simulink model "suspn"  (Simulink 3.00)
settings: Solver=ode45  SolverMode=SingleTasking  StartTime=0.0  StopTime=10  MaxStep=0.01  RelTol=1e-3  AbsTol=1e-6
PreLoadFcn:
  | suspdat
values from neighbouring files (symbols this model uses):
  cf = 2500    [suspdat.m]
  cr = 2000    [suspdat.m]
  Iyy = 2100    [suspdat.m]
  kf = 28000    [suspdat.m]
  kr = 21000    [suspdat.m]
  Lf = 0.9    [suspdat.m]
  Lr = 1.2    [suspdat.m]
  Mb = 1200    [suspdat.m]

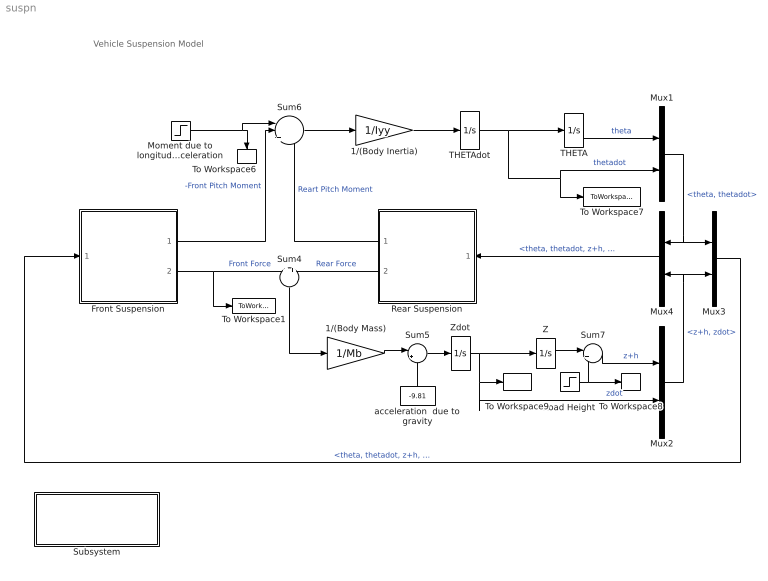
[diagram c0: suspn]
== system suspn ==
  note: Vehicle Suspension Model
  1/(Body Inertia) : Gain  Gain=1/Iyy  SaturateOnIntegerOverflow=on
  1/(Body Mass) : Gain  Gain=1/Mb  SaturateOnIntegerOverflow=on
  Front Suspension : Subsystem  mask(half-car suspension){K=kf, C=cf, L=-Lf}
      mask prompts: K "Stiffness = spring rate:"; C "Damping rate:"; L "Moment arm:"
      mask help: Half-Car Suspension The spring and damping rates for an individual wheel are entered below. Their combined effect as applied to two wheels at the specified distance from the center of mass is computed. The distance should be specified as positive if the subsystem is oriented such that increasing z corresponds to increasing theta, negative otherwise.
  Moment due to longitudinal vehicle acceleration : Step  Time=3  Before=0  After=100  SampleTime=0
  Mux1 : Mux  Inputs=2
  Mux2 : Mux  Inputs=2
  Mux3 : Mux  Inputs=2
  Mux4 : Mux  Orientation=left  Inputs=2
  Rear Suspension : Subsystem  Orientation=left  mask(half-car suspension){K=kr, C=cr, L=Lr}
      mask prompts: K "Stiffness = spring rate:"; C "Damping rate:"; L "Moment arm:"
      mask help: Half-Car Suspension The spring and damping rates for an individual wheel are entered below. Their combined effect as applied to two wheels at the specified distance from the center of mass is computed. The distance should be specified as positive if the subsystem is oriented such that increasing z corresponds to increasing theta, negative otherwise.
  Road Height : Step  Time=7  Before=0  After=0.01  SampleTime=0
  Subsystem : Subsystem
  Sum4 : Sum  Orientation=down  Inputs=++  SaturateOnIntegerOverflow=on
  Sum5 : Sum  Inputs=|++  SaturateOnIntegerOverflow=on
  Sum6 : Sum  Inputs=||+++  SaturateOnIntegerOverflow=on
  Sum7 : Sum  Inputs=|++  SaturateOnIntegerOverflow=on
  THETA : Integrator  ExternalReset=none  InitialConditionSource=internal  InitialCondition=-8.7e-20  LimitOutput=off  UpperSaturationLimit=inf  LowerSaturationLimit=-inf  ShowSaturationPort=off  ShowStatePort=off  AbsoluteTolerance=auto
  THETAdot : Integrator  ExternalReset=none  InitialConditionSource=internal  InitialCondition=8.04e-28  LimitOutput=off  UpperSaturationLimit=inf  LowerSaturationLimit=-inf  ShowSaturationPort=off  ShowStatePort=off  AbsoluteTolerance=auto
  To Workspace1 : ToWorkspace  VariableName=ForceF  SampleTime=0.01  SaveFormat=Matrix
  To Workspace6 : ToWorkspace  VariableName=Y  SampleTime=0.01  SaveFormat=Matrix
  To Workspace7 : ToWorkspace  VariableName=THETAdot  SampleTime=0.01  SaveFormat=Matrix
  To Workspace8 : ToWorkspace  VariableName=h  SampleTime=0.01  SaveFormat=Matrix
  To Workspace9 : ToWorkspace  VariableName=Zdot  SampleTime=0.01  SaveFormat=Matrix
  Z : Integrator  ExternalReset=none  InitialConditionSource=internal  InitialCondition=-0.12  LimitOutput=off  UpperSaturationLimit=inf  LowerSaturationLimit=-inf  ShowSaturationPort=off  ShowStatePort=off  AbsoluteTolerance=auto
  Zdot : Integrator  ExternalReset=none  InitialConditionSource=internal  InitialCondition=0  LimitOutput=off  UpperSaturationLimit=inf  LowerSaturationLimit=-inf  ShowSaturationPort=off  ShowStatePort=off  AbsoluteTolerance=auto
  acceleration  due to gravity : Constant  Orientation=up  Value=-9.81
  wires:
  Front Suspension/2(Vertical Force) -> Sum4/1, To Workspace1/1  "Front Force"
  Rear Suspension/2(Vertical Force) -> Sum4/2  "Rear Force"
  Sum4/1 -> 1/(Body Mass)/1
  Mux1/1 -> Mux3/1, Mux4/1  "<theta, thetadot>"
  Mux3/1 -> Front Suspension/1(THETA THETAdot Z Zdot)  "<theta, thetadot, z+h, zdot>"
  Mux4/1 -> Rear Suspension/1(THETA THETAdot Z Zdot)  "<theta, thetadot, z+h, zdot>"
  Sum5/1 -> Zdot/1
  acceleration  due to gravity/1 -> Sum5/2
  1/(Body Mass)/1 -> Sum5/1
  Z/1 -> Sum7/1
  Sum7/1 -> Mux2/1  "z+h"
  Zdot/1 -> Z/1, Mux2/2, To Workspace9/1  "zdot"
  Road Height/1 -> Sum7/2, To Workspace8/1
  Mux2/1 -> Mux3/2, Mux4/2  "<z+h, zdot>"
  Moment due to longitudinal vehicle acceleration/1 -> To Workspace6/1, Sum6/1
  Sum6/1 -> 1/(Body Inertia)/1
  Rear Suspension/1(pitch Torque) -> Sum6/3  "Reart Pitch Moment"
  Front Suspension/1(pitch Torque) -> Sum6/2  "-Front Pitch Moment"
  1/(Body Inertia)/1 -> THETAdot/1
  THETA/1 -> Mux1/1  "theta"
  THETAdot/1 -> THETA/1, To Workspace7/1, Mux1/2  "thetadot"

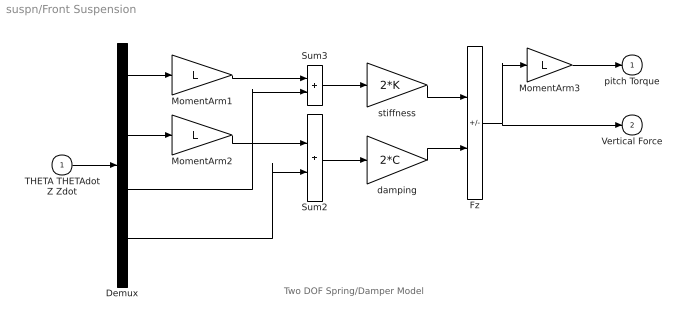
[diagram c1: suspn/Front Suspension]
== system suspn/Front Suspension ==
  note: Two DOF Spring/Damper Model
  THETA THETAdot Z Zdot : Inport  Port=1  PortWidth=-1  SampleTime=-1  DataType=auto
  Demux : Demux  Outputs=4
  Fz : Sum  Inputs=--  SaturateOnIntegerOverflow=on
  MomentArm1 : Gain  Gain=L  SaturateOnIntegerOverflow=on
  MomentArm2 : Gain  Gain=L  SaturateOnIntegerOverflow=on
  MomentArm3 : Gain  Gain=L  SaturateOnIntegerOverflow=on
  Sum2 : Sum  Inputs=++  SaturateOnIntegerOverflow=on
  Sum3 : Sum  Inputs=++  SaturateOnIntegerOverflow=on
  damping : Gain  Gain=2*C  SaturateOnIntegerOverflow=on
  stiffness : Gain  Gain=2*K  SaturateOnIntegerOverflow=on
  pitch Torque : Outport  Port=1  InitialOutput=0
  Vertical Force : Outport  Port=2  InitialOutput=0
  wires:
  Sum2/1 -> damping/1
  Sum3/1 -> stiffness/1
  THETA THETAdot Z Zdot/1 -> Demux/1
  damping/1 -> Fz/2
  stiffness/1 -> Fz/1
  Fz/1 -> Vertical Force/1, MomentArm3/1
  MomentArm3/1 -> pitch Torque/1
  Demux/1 -> MomentArm1/1
  Demux/2 -> MomentArm2/1
  Demux/3 -> Sum3/2
  MomentArm1/1 -> Sum3/1
  MomentArm2/1 -> Sum2/1
  Demux/4 -> Sum2/2

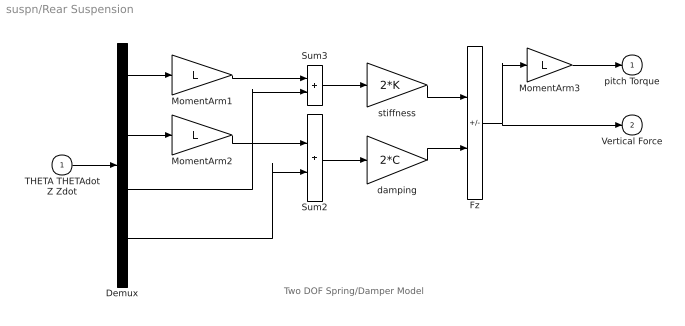
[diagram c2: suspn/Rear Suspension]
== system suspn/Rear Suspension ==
  note: Two DOF Spring/Damper Model
  THETA THETAdot Z Zdot : Inport  Port=1  PortWidth=-1  SampleTime=-1  DataType=auto
  Demux : Demux  Outputs=4
  Fz : Sum  Inputs=--  SaturateOnIntegerOverflow=on
  MomentArm1 : Gain  Gain=L  SaturateOnIntegerOverflow=on
  MomentArm2 : Gain  Gain=L  SaturateOnIntegerOverflow=on
  MomentArm3 : Gain  Gain=L  SaturateOnIntegerOverflow=on
  Sum2 : Sum  Inputs=++  SaturateOnIntegerOverflow=on
  Sum3 : Sum  Inputs=++  SaturateOnIntegerOverflow=on
  damping : Gain  Gain=2*C  SaturateOnIntegerOverflow=on
  stiffness : Gain  Gain=2*K  SaturateOnIntegerOverflow=on
  pitch Torque : Outport  Port=1  InitialOutput=0
  Vertical Force : Outport  Port=2  InitialOutput=0
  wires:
  Demux/4 -> Sum2/2
  MomentArm2/1 -> Sum2/1
  MomentArm1/1 -> Sum3/1
  Demux/3 -> Sum3/2
  Demux/2 -> MomentArm2/1
  Demux/1 -> MomentArm1/1
  MomentArm3/1 -> pitch Torque/1
  Fz/1 -> MomentArm3/1, Vertical Force/1
  stiffness/1 -> Fz/1
  damping/1 -> Fz/2
  THETA THETAdot Z Zdot/1 -> Demux/1
  Sum3/1 -> stiffness/1
  Sum2/1 -> damping/1

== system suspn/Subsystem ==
